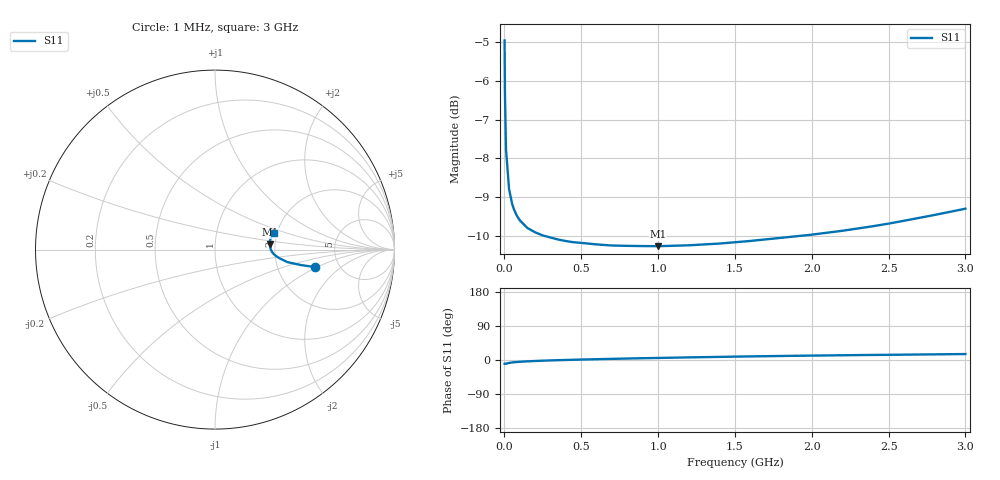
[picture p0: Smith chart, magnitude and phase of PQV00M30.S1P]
! SIEMENS Small Signal Semiconductors
! BAR64-04
! Si PIN Diode in SOT23 (2 diodes in series, pin 3 open)
! IF = 0.3 mA
! S-Parameters:  July  1992
# GHz  S  MA  R  50
!  f  S11
! GHz  MAG  ANG
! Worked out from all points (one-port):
!   33 points, 1 MHz to 3 GHz, reference 50 ohm
!   lowest |S11| = -10.3 dB at 1 GHz (marker M1), VSWR 1.88, Z = 93.6 + j5.96 ohm
!   |S11| at or under -10 dB: 251.9 MHz to 1.942 GHz (1.69 GHz wide, 154 % of centre)
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0.001  0.5657 -9.9
0.003  0.4857 -10.2
0.01  0.4093 -9.8
0.03  0.3633 -7.7
0.05  0.3475 -6.5
0.06  0.3427 -6.1
0.08  0.3357 -5.3
0.1  0.3309 -4.7
0.15  0.3234 -3.5
0.2  0.3193 -2.6
0.25  0.3163 -1.8
0.35  0.3125 -0.5
0.4  0.3111 0.1
0.45  0.31 0.6
0.5  0.3094 1.2
0.6  0.308 2.1
0.7  0.307 3.0
0.8  0.3067 3.9
1  0.3064 5.4
1.2  0.3072 6.9
1.4  0.3088 8.2
1.6  0.3112 9.5
2  0.3171 11.6
2.2  0.3208 12.5
2.4  0.3252 13.4
2.5  0.3277 13.7
2.8  0.3363 14.9
3  0.3426 15.7
